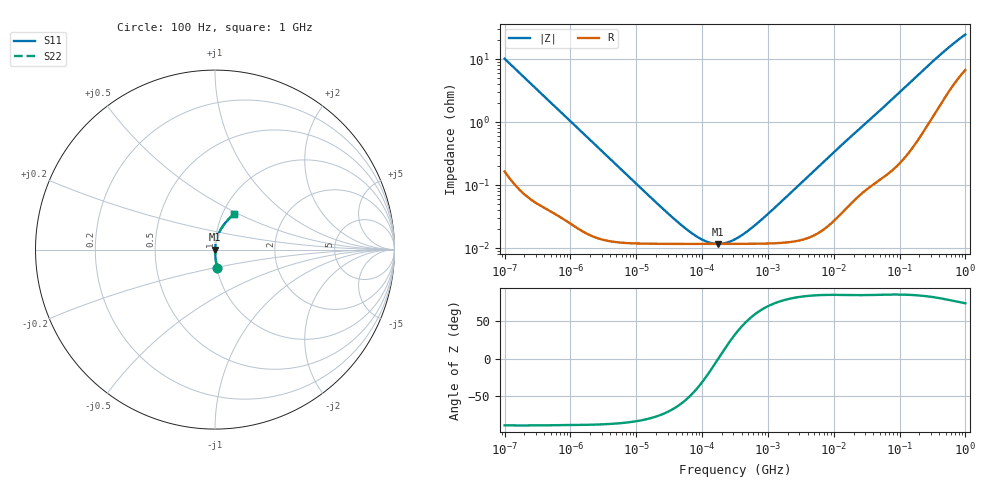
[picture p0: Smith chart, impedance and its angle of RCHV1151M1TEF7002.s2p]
! RCHV1151M1TEF7002  S-PARAMETER MODEL  (AEC-Q200 qualified)
! Model Generated by ELNA Corporation (http://www.ty-top.com)
! Version 1.0
! ELNA Control No. 240229
! Copyright (c) 2024 ELNA CO.,LTD. All Rights Reserved.
! Products Name : CONDUCTIVE POLYMER HYBRID ALUMINUM ELECTROLYTIC CAPACITORS
! Characteristics :
!  Capacitance  :  150uF  ,  Rated voltage  :  25V
!  Operating Temp. Range  :  -55 to +105 degC  ,  Endurance  :  5000hr at 105 degC
!  Dimension D  :  8mm  ,  Dimension L  :  8.7mm
! Frequency Range : 100Hz - 1GHz
! External Node Assignments :
!  1  o---| |---o  2
# MHz S RI R 50
!Freq[MHz].  S11 Real  S11 Imag  S21 Real  S21 Imag  S12 Real  S12 Imag  S22 Real  S22 Imag
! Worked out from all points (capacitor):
!   401 points, 100 Hz to 1 GHz, reference 50 ohm
!   read as one part in series: C = 155 uF near 108 Hz
!   lowest |Z| = 11.6 mohm at 172.8 kHz (marker M1)
!   series resonance near 176.1 kHz, so ESL is about 5.3 nH
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0.0001  0.012 -0.1011  0.988 0.1011  0.988 0.1011  0.012 -0.1011
0.000113  0.00953 -0.0898  0.9905 0.0898  0.9905 0.0898  0.00953 -0.0898
0.000309  0.00161 -0.0332  0.9984 0.0332  0.9984 0.0332  0.00161 -0.0332
0.001488  0.000236 -0.00701  0.9998 0.00701  0.9998 0.00701  0.000236 -0.00701
0.022131  0.000117 -0.000466  0.9999 0.000466  0.9999 0.000466  0.000117 -0.000466
0.045709  0.000116 -0.000214  0.9999 0.000214  0.9999 0.000214  0.000116 -0.000214
0.077179  0.000116 -0.00011  0.9999 0.00011  0.9999 0.00011  0.000116 -0.00011
0.098288  0.000116 -7.34e-05  0.9999 7.34e-05  0.9999 7.34e-05  0.000116 -7.34e-05
0.120226  0.000116 -4.65e-05  0.9999 4.65e-05  0.9999 4.65e-05  0.000116 -4.65e-05
0.172783  0.000116 -2.26e-06  0.9999 2.26e-06  0.9999 2.26e-06  0.000116 -2.26e-06
0.229087  0.000116 3.17e-05  0.9999 -3.17e-05  0.9999 -3.17e-05  0.000116 3.17e-05
0.316228  0.000116 7.37e-05  0.9999 -7.37e-05  0.9999 -7.37e-05  0.000116 7.37e-05
0.473151  0.000116 0.000138  0.9999 -0.000138  0.9999 -0.000138  0.000116 0.000138
0.767361  0.000117 0.000246  0.9999 -0.000246  0.9999 -0.000246  0.000117 0.000246
1.462177  0.00012 0.000487  0.9999 -0.000487  0.9999 -0.000487  0.00012 0.000487
4.704354  0.000156 0.00158  0.9998 -0.00158  0.9998 -0.00158  0.000156 0.00158
12.8825  0.000367 0.00424  0.9996 -0.00424  0.9996 -0.00424  0.000367 0.00424
69.9842  0.00201 0.021  0.998 -0.021  0.998 -0.021  0.00201 0.021
176.8072  0.00733 0.0516  0.9927 -0.0516  0.9927 -0.0516  0.00733 0.0516
395.8221  0.029 0.1071  0.971 -0.1071  0.971 -0.1071  0.029 0.1071
668.3439  0.0655 0.1584  0.9345 -0.1584  0.9345 -0.1584  0.0655 0.1584
1000  0.1085 0.2002  0.8915 -0.2002  0.8915 -0.2002  0.1085 0.2002
